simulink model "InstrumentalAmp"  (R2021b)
settings: Solver=VariableStepAuto  StartTime=0.0  StopTime=10.0  RelTol=1e-3
libraries: fl_lib x19, nesl_utility x4

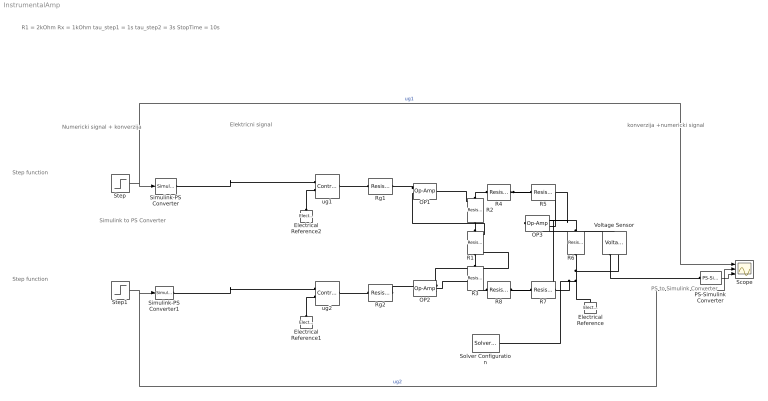
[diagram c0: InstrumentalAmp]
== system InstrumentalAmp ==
  note: Elektricni signal
  note: konverzija +numericki signal
  note: Numericki signal + konverzija
  note: PS to Simulink Converter
  note: Simulink to PS Converter
  note: Step function
  note: Step function
  note: R1 = 2kOhm Rx = 1kOhm tau_step1 = 1s tau_step2 = 3s StopTime = 10s
  Electrical Reference : fl_lib/Electrical/Electrical Elements/Electrical Reference
  Electrical Reference1 : fl_lib/Electrical/Electrical Elements/Electrical Reference
  Electrical Reference2 : fl_lib/Electrical/Electrical Elements/Electrical Reference
  OP1 : fl_lib/Electrical/Electrical Elements/Op-Amp  outI_specify=off  outI_priority=None  outI=0 A  outI_nominal_specify=off  outI_nominal_unit=A  outI_nominal_value=1
  OP2 : fl_lib/Electrical/Electrical Elements/Op-Amp  outI_specify=off  outI_priority=None  outI=0 A  outI_nominal_specify=off  outI_nominal_unit=A  outI_nominal_value=1
  OP3 : fl_lib/Electrical/Electrical Elements/Op-Amp  outI_specify=off  outI_priority=None  outI=0 A  outI_nominal_specify=off  outI_nominal_unit=A  outI_nominal_value=1
  PS-Simulink Converter : nesl_utility/PS-Simulink Converter  PhysicalDomain=network_engine_domain  SubClassName=ps_output  LeftPortType=input  RightPortType=output  PseudoPeriodic=off  Frequencies=[]  Unit=1  AffineConversion=off
  R1 : fl_lib/Electrical/Electrical Elements/Resistor  R=2000 Ohm  i_specify=off  i_priority=None  i=0 A  i_nominal_specify=off  i_nominal_unit=A  i_nominal_value=1  v_specify=off  v_priority=None  v=0 V  v_nominal_specify=off  v_nominal_unit=V  v_nominal_value=1
  R{2..8} (7 alike) : fl_lib/Electrical/Electrical Elements/Resistor  R=1000 Ohm  i_specify=off  i_priority=None  i=0 A  i_nominal_specify=off  i_nominal_unit=A  i_nominal_value=1  v_specify=off  v_priority=None  v=0 V  v_nominal_specify=off  v_nominal_unit=V  v_nominal_value=1
  Rg1 : fl_lib/Electrical/Electrical Elements/Resistor  R=2000 Ohm  i_specify=off  i_priority=None  i=0 A  i_nominal_specify=off  i_nominal_unit=A  i_nominal_value=1  v_specify=off  v_priority=None  v=0 V  v_nominal_specify=off  v_nominal_unit=V  v_nominal_value=1
  Rg2 : fl_lib/Electrical/Electrical Elements/Resistor  R=2000 Ohm  i_specify=off  i_priority=None  i=0 A  i_nominal_specify=off  i_nominal_unit=A  i_nominal_value=1  v_specify=off  v_priority=None  v=0 V  v_nominal_specify=off  v_nominal_unit=V  v_nominal_value=1
  Scope : Scope  NumInputPorts=3
  Simulink-PS Converter : nesl_utility/Simulink-PS Converter  PhysicalDomain=network_engine_domain  SubClassName=ps_input  LeftPortType=input  RightPortType=output  PseudoPeriodic=off  Frequencies=[]  NoiseDistribution=none  NoiseParameters=[]  Unit=1  AffineConversion=off  FilteringAndDerivatives=provide  SimscapeFilterOrder=1  InputFilterTimeConstant=0.001  UdotUserProvided=0
  Simulink-PS Converter1 : nesl_utility/Simulink-PS Converter  PhysicalDomain=network_engine_domain  SubClassName=ps_input  LeftPortType=input  RightPortType=output  PseudoPeriodic=off  Frequencies=[]  NoiseDistribution=none  NoiseParameters=[]  Unit=1  AffineConversion=off  FilteringAndDerivatives=provide  SimscapeFilterOrder=1  InputFilterTimeConstant=0.001  UdotUserProvided=0
  Solver Configuration : nesl_utility/Solver Configuration  PhysicalDomain=network_engine_domain  SubClassName=solver  LeftPortType=input  RightPortType=generic  Tones=[]  Harmonics=[]  SimulateNoise=off  Profile=off  UseLocalSampling=off  EnableSwitchedLinearOptims=on  FrequencyDomain=off  UseCCode=off  RelTol=0.001  AbsTol=1e-06  MinStep=1e-09  ToWorkspace=off  RevertToSquareIcSolve=off  NumHomotopyIterations=100  PhasorMode=off  PhasorModeNumHarmonics=1  DoDC=off  ResidualTolerance=1e-09  UseLocalSolver=off  LocalSolverChoice=NE_BACKWARD_EULER_ADVANCER  LocalSolverSampleTime=0.001  DoFixedCost=off  MaxNonlinIter=3  MaxModeIter=2  ComputeImpulses=off  ImpulseIterations=2  LinearAlgebra=Sparse  EquationFormulation=NE_TIME_EF  DelaysMemoryBudget=1024  AutomaticFiltering=on  FilteringTimeConstant=0.001  PartitionStorageMethod=AS_NEEDED  PartitionMemoryBudget=1024  PartitionMethod=FAST
  Step : Step  SampleTime=0
  Step1 : Step  Time=3  SampleTime=0
  Voltage Sensor : fl_lib/Electrical/Electrical Sensors/Voltage Sensor
  ug1 : fl_lib/Electrical/Electrical Sources/Controlled Voltage Source
  ug2 : fl_lib/Electrical/Electrical Sources/Controlled Voltage Source
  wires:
  Step/1 -> Scope/1, Simulink-PS Converter/1  "ug1"
  Step1/1 -> Scope/2, Simulink-PS Converter1/1  "ug2"
  PS-Simulink Converter/1 -> Scope/3
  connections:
  R1/LConn1 -- OP1/LConn2 -- R2/RConn1
  R1/RConn1 -- OP2/LConn2 -- R3/LConn1
  Rg2/RConn1 -- OP2/LConn1
  OP1/LConn1 -- Rg1/RConn1
  R3/RConn1 -- OP2/RConn1 -- R8/LConn1
  R8/RConn1 -- OP3/LConn1 -- R7/LConn1
  R2/LConn1 -- OP1/RConn1 -- R4/LConn1
  R4/RConn1 -- OP3/LConn2 -- R5/LConn1
  OP3/RConn1 -- R6/LConn1 -- Voltage Sensor/LConn1 -- R5/RConn1
  R6/RConn1 -- Voltage Sensor/RConn2 -- Electrical Reference/LConn1 -- Solver Configuration/RConn1 -- R7/RConn1
  Electrical Reference1/LConn1 -- ug2/RConn2
  Electrical Reference2/LConn1 -- ug1/RConn2
  ug1/LConn1 -- Rg1/LConn1
  ug2/LConn1 -- Rg2/LConn1
  Simulink-PS Converter/RConn1 -- ug1/RConn1
  Simulink-PS Converter1/RConn1 -- ug2/RConn1
  Voltage Sensor/RConn1 -- PS-Simulink Converter/LConn1
